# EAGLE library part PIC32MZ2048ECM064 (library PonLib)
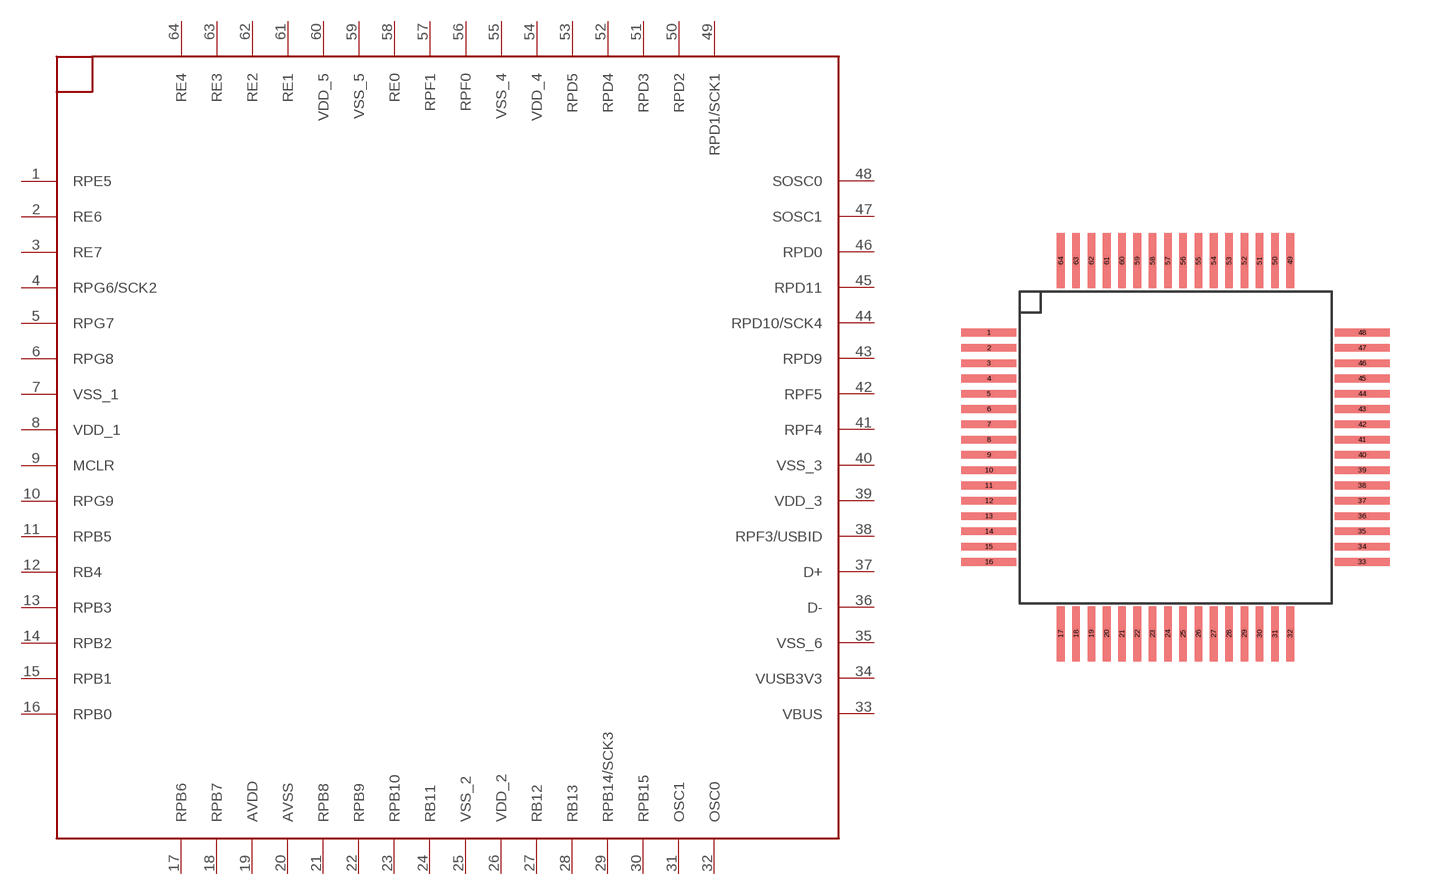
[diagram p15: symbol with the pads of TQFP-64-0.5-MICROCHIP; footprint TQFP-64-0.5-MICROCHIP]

Designator prefix -

## PIC32MZ2048ECM064  [TQFP-64-0.5-MICROCHIP]
1  RPE5
2  RE6
3  RE7
4  RPG6/SCK2
5  RPG7
6  RPG8
7  VSS_1
8  VDD_1
9  MCLR
10  RPG9
11  RPB5
12  RB4
13  RPB3
14  RPB2
15  RPB1
16  RPB0
17  RPB6
18  RPB7
19  AVDD
20  AVSS
21  RPB8
22  RPB9
23  RPB10
24  RB11
25  VSS_2
26  VDD_2
27  RB12
28  RB13
29  RPB14/SCK3
30  RPB15
31  OSC1
32  OSC0
33  VBUS
34  VUSB3V3
35  VSS_6
36  D-
37  D+
38  RPF3/USBID
39  VDD_3
40  VSS_3
41  RPF4
42  RPF5
43  RPD9
44  RPD10/SCK4
45  RPD11
46  RPD0
47  SOSC1
48  SOSC0
49  RPD1/SCK1
50  RPD2
51  RPD3
52  RPD4
53  RPD5
54  VDD_4
55  VSS_4
56  RPF0
57  RPF1
58  RE0
59  VSS_5
60  VDD_5
61  RE1
62  RE2
63  RE3
64  RE4

## Footprint TQFP-64-0.5-MICROCHIP (pad centres in mm)
smd 1.8 x 0.25: 1 -6.1,3.75; 2 -6.1,3.25; 3 -6.1,2.75; 4 -6.1,2.25; 5 -6.1,1.75; 6 -6.1,1.25; 7 -6.1,0.75; 8 -6.1,0.25; 9 -6.1,-0.25; 10 -6.1,-0.75; 11 -6.1,-1.25; 12 -6.1,-1.75; 13 -6.1,-2.25; 14 -6.1,-2.75; 15 -6.1,-3.25; 16 -6.1,-3.75; 33 6.1,-3.75; 34 6.1,-3.25; 35 6.1,-2.75; 36 6.1,-2.25; 37 6.1,-1.75; 38 6.1,-1.25; 39 6.1,-0.75; 40 6.1,-0.25; 41 6.1,0.25; 42 6.1,0.75; 43 6.1,1.25; 44 6.1,1.75; 45 6.1,2.25; 46 6.1,2.75; 47 6.1,3.25; 48 6.1,3.75
smd 0.25 x 1.8: 17 -3.75,-6.1; 18 -3.25,-6.1; 19 -2.75,-6.1; 20 -2.25,-6.1; 21 -1.75,-6.1; 22 -1.25,-6.1; 23 -0.75,-6.1; 24 -0.25,-6.1; 25 0.25,-6.1; 26 0.75,-6.1; 27 1.25,-6.1; 28 1.75,-6.1; 29 2.25,-6.1; 30 2.75,-6.1; 31 3.25,-6.1; 32 3.75,-6.1; 49 3.75,6.1; 50 3.25,6.1; 51 2.75,6.1; 52 2.25,6.1; 53 1.75,6.1; 54 1.25,6.1; 55 0.75,6.1; 56 0.25,6.1; 57 -0.25,6.1; 58 -0.75,6.1; 59 -1.25,6.1; 60 -1.75,6.1; 61 -2.25,6.1; 62 -2.75,6.1; 63 -3.25,6.1; 64 -3.75,6.1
